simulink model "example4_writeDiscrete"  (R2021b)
settings: Solver=FixedStepDiscrete  StartTime=0.0  StopTime=inf  FixedStep=0.8  RelTol=1e-3
libraries: ModbusServerLib x3

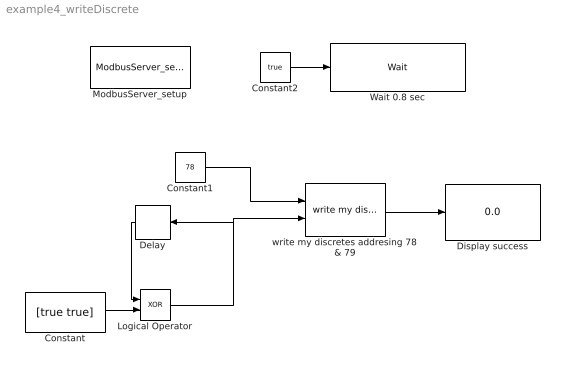
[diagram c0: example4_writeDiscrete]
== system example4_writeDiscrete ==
  Constant : Constant  Value=[true true]
  Constant1 : Constant  Value=78
  Constant2 : Constant  Value=true
  Delay : Delay  DelayLength=1  InitialCondition=[false false]
  Display success : Display
  Logical Operator : Logic  Operator=XOR  AllPortsSameDT=off  OutDataTypeStr=boolean
  ModbusServer_setup : ModbusServerLib/ModbusServer_setup  g1_cmbPortName="\"COM5\""  g2_cmbModbusType="\"Modbus TCP\""  g3_chkIgnoreServerID=off  g4_ObjectID=0  g5_ServerID=1  g30_TCPPort=502  g6_chkSupportDINCoil1to4=on  g7_HoldingRegsSeg1to4=[ 1,30 ; 35, 56]  g8_InputRegsSeg1to4=[1 44; 78 89]  g9_CoilSeg1to4=[1 44; 78 89]  g10_DiscreteSeg1to4=[1 44; 78 89]  g11_chkUseHoldingRegstoReplace1to4=off  g12_chkEnableWD1to4=off  g13_chkUseReadonlyRegs4WD1to4=off  g14_WDAddr1to4=1  g15_cmbWDType1to4=0  g16_WDPeriod1to4=20  g17_WDPreset1to4=20  g18_chkSupportDINCoil5=on  g19_HoldingRegsSeg5=[ 1,30 ; 35, 56]  g20_InputRegsSeg5=[1 44; 78 89]  g21_CoilSeg5=[1 44; 78 89]  g22_DiscreteSeg5=[1 44; 78 89]  g23_chkUseHoldingRegstoReplace5=off  g24_chkEnableWD5=off  g25_chkUseReadonlyRegs4WD5=off  g26_WDAddr5=1  g27_cmbWDType5=0  g28_WDPeriod5=20  g29_WDPreset5=20
  Wait 0.8 sec : ModbusServerLib/Wait  Waitms=800
  write my discretes addresing 78 & 79 : ModbusServerLib/write my discretes  g_ObjID=0  g_DeviceNo=1
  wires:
  Constant1/1 -> write my discretes addresing 78 & 79/1
  Constant2/1 -> Wait 0.8 sec/1
  write my discretes addresing 78 & 79/1 -> Display success/1
  Delay/1 -> Logical Operator/1
  Constant/1 -> Logical Operator/2
  Logical Operator/1 -> Delay/1, write my discretes addresing 78 & 79/2
